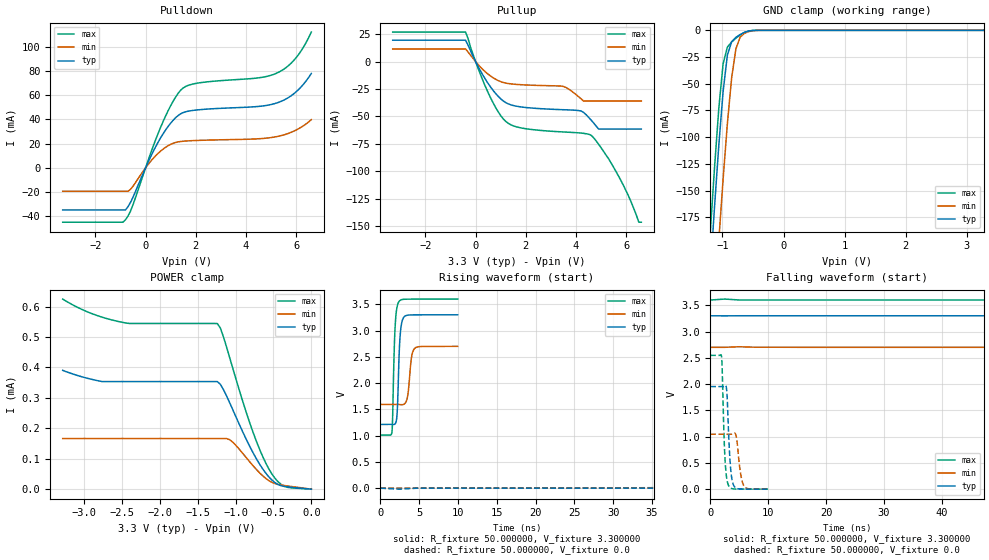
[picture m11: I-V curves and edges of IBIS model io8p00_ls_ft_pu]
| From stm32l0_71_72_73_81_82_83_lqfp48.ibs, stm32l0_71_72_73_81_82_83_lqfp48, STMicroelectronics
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|   Model io8p00_ls_ft_pu
[Model]  io8p00_ls_ft_pu
Model_type I/O
Polarity   Non-Inverting
Enable   Active-Low
Vinl =   0.990000V
Vinh =   2.310000V
Vmeas =  1.650000V
Cref =   50.000000pF
Rref =   100.000000M
Vref =   0.0V
C_comp   4.606100pF   4.563500pF   4.706200pF
[Temperature Range]   25.000000   0.125000k   -40.000000
[Pullup Reference]   3.300000V   2.700000V   3.600000V
[Pulldown Reference]   0.0V   0.0V   0.0V
[POWER Clamp Reference]   3.300000V   2.700000V   3.600000V
[GND Clamp Reference]   0.0V   0.0V   0.0V
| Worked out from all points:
|   slope of the pulldown table from 0 to 0.495 V, typ, clamps not added: 23.6 ohm
|   slope of the pullup table from 0 to 0.495 V, typ, clamps not added: 24.9 ohm
|   GND clamp passes 1 mA (typ) near -0.59 V on its own axis
|   rising waveform, R_fixture 50.000000, V_fixture 3.300000: 20-80 % time 316ps typ, 427ps min, 298ps max; typ from 1.21 V to 3.3 V
|   rising waveform, R_fixture 50.000000, V_fixture 0.0: 20-80 % time 204ns typ, 424ns min, 100ns max; typ from 0.001 V to 1.95 V
|   falling waveform, R_fixture 50.000000, V_fixture 3.300000: 20-80 % time 194ns typ, 379ns min, 107ns max; typ from 3.3 V to 1.21 V
|   falling waveform, R_fixture 50.000000, V_fixture 0.0: 20-80 % time 526ps typ, 689ps min, 462ps max; typ from 1.95 V to 0.001 V
[Pulldown]
|Voltage   I(typ)   I(min)   I(max)
-3.3V     -34.78mA   -19.34mA   -44.89mA
-900mV    -34.78mA   -19.34mA   -44.89mA
-800mV    -34.78mA   -19.34mA   -42.84mA
-600mV    -28.56mA   -17.8mA    -35.75mA
100mV     4.638mA    2.744mA    6.076mA
600mV     24.8mA     13.84mA    33.52mA
1V        36.93mA    19.39mA    51.35mA
1.4V      44.67mA    21.76mA    64.17mA
2V        47.71mA    22.58mA    69.7mA
5.2V      53.42mA    25.71mA    78.01mA
6V        62.87mA    31.27mA    91.1mA
6.6V      77.92mA    39.75mA    112.1mA
[Pullup]
|Voltage   I(typ)   I(min)   I(max)
-3.3V     19.51mA    11.53mA    26.92mA
-400mV    19.51mA    11.53mA    26.92mA
400mV     -16.48mA   -9.566mA   -23.24mA
1.1V      -35.89mA   -19.06mA   -52.21mA
1.7V      -41.02mA   -20.95mA   -60.01mA
3.5V      -43.94mA   -22.7mA    -64.24mA
4.2V      -45.07mA   -33.96mA   -65.24mA
4.6V      -53.37mA   -35.99mA   -67.22mA
4.9V      -61.63mA   -35.99mA   -75.49mA
5.8V      -61.63mA   -35.99mA   -109.1mA
6.5V      -61.63mA   -35.99mA   -146.6mA
6.6V      -61.63mA   -35.99mA   -146.6mA
[GND_clamp]
|Voltage   I(typ)   I(min)   I(max)
-3.3V     -2.276A    -2.356A    -2.25A
-1.2V     -226mA     -318.7mA   -189.2mA
-1.13V    -164.9mA   -256.6mA   -128.3mA
-1.06V    -107.5mA   -196.5mA   -72.78mA
-990mV    -57.32mA   -139.4mA   -31.39mA
-920mV    -23.22mA   -87.32mA   -15.73mA
-850mV    -10.58mA   -44.45mA   -10.94mA
-780mV    -6.539mA   -17.25mA   -7.356mA
-710mV    -3.933mA   -6.349mA   -4.308mA
-640mV    -1.955mA   -2.79mA    -1.975mA
-360mV    -2.06uA    -16.21uA   -459.5nA
3.28V     0A         0A         0A
[POWER_clamp]
|Voltage   I(typ)   I(min)   I(max)
-3.28V    390.5uA    166.4uA    624.7uA
-2.76V    353.6uA    166.4uA    565.1uA
-2.44V    353.6uA    166.4uA    545.7uA
-1.24V    353.6uA    166.4uA    544.1uA
-1.2V     344.6uA    166.4uA    529.4uA
-1.16V    327.5uA    166.4uA    501.1uA
-1.04V    263.2uA    155.2uA    400.5uA
-760mV    115.6uA    74.53uA    180.9uA
-560mV    40.33uA    28.04uA    66.46uA
-440mV    15.38uA    15.6uA     24.56uA
-360mV    9.136uA    12.12uA    10.1uA
0V        0A         0A         0A
[Ramp]
| variable   typ   min   max
dV/dt_r  1.17099/0.20424u   0.60212/0.42558u   1.52743/0.10012u
dV/dt_f  1.24968/0.19373u   0.62364/0.37971u   1.55250/0.10680u
R_load = 50.000000
[Rising Waveform]
R_fixture= 50.000000
V_fixture= 3.300000
V_fixture_min= 2.700000
V_fixture_max= 3.600000
|time   V(typ)   V(min)   V(max)
0s        1.214V     1.595V     1.012V
1.502ns   1.214V     1.595V     1.068V
1.902ns   1.224V     1.595V     3.038V
2.162ns   1.409V     1.595V     3.449V
2.362ns   2.239V     1.593V     3.541V
2.643ns   3.033V     1.59V      3.582V
3.103ns   3.266V     1.604V     3.595V
3.524ns   3.292V     1.751V     3.597V
4.404ns   3.298V     2.657V     3.598V
9.97ns    3.3V       2.7V       3.599V
[Rising Waveform]
R_fixture= 50.000000
V_fixture= 0.0
V_fixture_min= 0.0
V_fixture_max= 0.0
|time   V(typ)   V(min)   V(max)
0s        1.146mV    1.863mV    784.1uV
52.55ns   5.274mV    4.548mV    119.7mV
95.1ns    61.92mV    4.577mV    820.9mV
140.1ns   292.6mV    8.089mV    1.578V
185.2ns   600.6mV    14.2mV     2.102V
265.3ns   1.137V     70.06mV    2.458V
387.9ns   1.647V     243.4mV    2.534V
535.5ns   1.871V     499.2mV    2.545V
853.4ns   1.948V     889.6mV    2.547V
1.246us   1.953V     1.046V     2.546V
[Falling Waveform]
R_fixture= 50.000000
V_fixture= 3.300000
V_fixture_min= 2.700000
V_fixture_max= 3.600000
|time   V(typ)   V(min)   V(max)
0s        3.3V       2.7V       3.599V
82.58ns   3.3V       2.7V       3.499V
145.1ns   3.215V     2.7V       2.61V
217.7ns   2.824V     2.696V     1.584V
255.3ns   2.57V      2.685V     1.249V
292.8ns   2.308V     2.662V     1.119V
402.9ns   1.63V      2.541V     1.039V
518ns     1.351V     2.347V     1.02V
845.8ns   1.232V     1.79V      1.012V
1.246us   1.214V     1.595V     1.012V
[Falling Waveform]
R_fixture= 50.000000
V_fixture= 0.0
V_fixture_min= 0.0
V_fixture_max= 0.0
|time   V(typ)   V(min)   V(max)
0s        1.953V     1.046V     2.546V
1.942ns   1.953V     1.046V     2.527V
2.523ns   1.965V     1.046V     622.1mV
2.843ns   1.871V     1.046V     206.6mV
3.123ns   1.173V     1.046V     79.61mV
3.544ns   359.9mV    1.046V     20.18mV
4.124ns   56.14mV    1.066V     4.521mV
4.525ns   16.4mV     982mV      2.852mV
5.746ns   1.922mV    75.99mV    1.647mV
9.97ns    1.146mV    1.863mV    784.1uV
